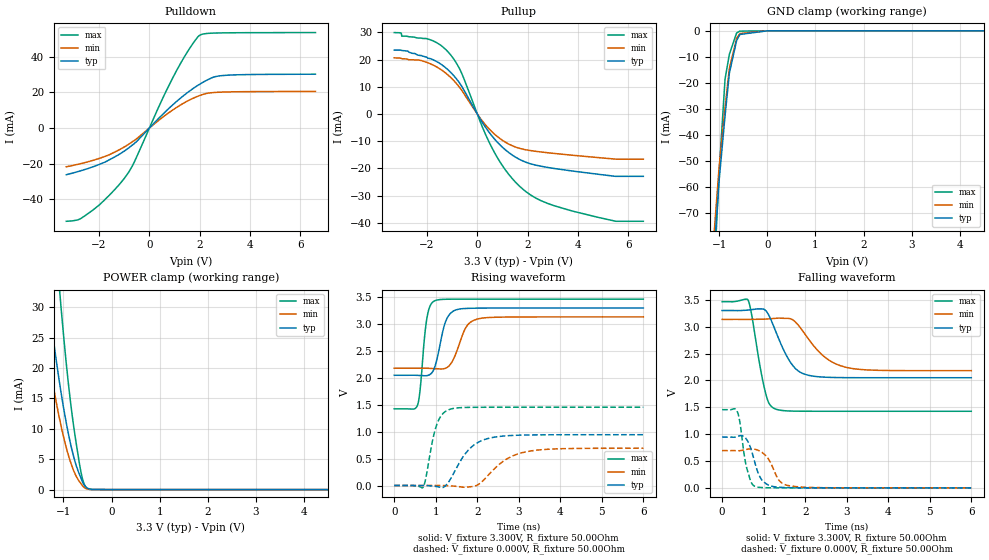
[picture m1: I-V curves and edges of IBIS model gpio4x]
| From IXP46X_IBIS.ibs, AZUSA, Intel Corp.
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[Model]   gpio4x
Model_type   I/O
Vinl = 800.000mV
Vinh = 2.000V
Vmeas = 1.500V
Cref = 0.000F
|   typ   min   max
C_comp   3.000pF   2.700pF   3.300pF
[Voltage Range]   3.300V   3.135V   3.465V
[Temperature Range]   25.0   110.0   -40.0
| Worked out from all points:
|   slope of the pulldown table from 0 to 0.495 V, typ, clamps not added: 68.7 ohm
|   slope of the pullup table from 0 to 0.495 V, typ, clamps not added: 70.3 ohm
|   POWER clamp passes 1 mA (typ) near -0.59 V on its own axis
|   falling waveform, V_fixture 3.300V, R_fixture 50.00Ohm: 20-80 % time 460ps typ, 667ps min, 278ps max; typ from 3.3 V to 2.05 V
|   rising waveform, V_fixture 3.300V, R_fixture 50.00Ohm: 20-80 % time 226ps typ, 291ps min, 146ps max; typ from 2.05 V to 3.3 V
|   rising waveform, V_fixture 0.000V, R_fixture 50.00Ohm: 20-80 % time 520ps typ, 669ps min, 242ps max; typ from 0 V to 0.944 V
|   falling waveform, V_fixture 0.000V, R_fixture 50.00Ohm: 20-80 % time 241ps typ, 274ps min, 183ps max; typ from 0.944 V to 0 V
[Pulldown]
|   Voltage   I(typ)   I(min)   I(max)
-3.3V     -26.23mA   -21.78mA   -52.39mA
-2.81V    -24.38mA   -20.3mA    -51.42mA
-2.245V   -21.81mA   -18.2mA    -46.09mA
-1.565V   -17.68mA   -14.82mA   -37.38mA
-910mV    -12.13mA   -9.924mA   -26.64mA
-605mV    -8.83mA    -7.087mA   -19.28mA
940mV     13.15mA    10.23mA    28.48mA
1.535V    20.1mA     15.3mA     43.29mA
1.99V     24.51mA    18.19mA    51.99mA
2.545V    28.53mA    19.9mA     53.28mA
2.875V    29.4mA     20.15mA    53.4mA
6.595V    30.22mA    20.54mA    53.58mA
[GND Clamp]
|   Voltage   I(typ)   I(min)   I(max)
-3.3V     -1.837A    -1.782A    -2.189A
-1.12V    -88.02mA   -80.79mA   -98.45mA
-1.005V   -57.96mA   -52.72mA   -55.07mA
-1V       -56.71mA   -51.74mA   -53.25mA
-880mV    -32.63mA   -29.48mA   -18.52mA
-790mV    -16.22mA   -14.39mA   -8.985mA
-640mV    -3.751mA   -2.926mA   -836.8uA
-575mV    -1.515mA   -1.11mA    -135.3uA
0V        -56.84nA   -17.58nA   -565.5pA
6.595V    0A         0A         0A
[Pullup]
|   Voltage   I(typ)   I(min)   I(max)
-3.3V     23.5mA     20.67mA    29.96mA
-1.775V   20.04mA    18.1mA     26.98mA
-1.055V   15.31mA    13.43mA    21.71mA
-630mV    10.36mA    8.892mA    15.17mA
215mV     -3.323mA   -2.738mA   -5.088mA
695mV     -9.323mA   -7.506mA   -14.38mA
1.25V     -14.19mA   -11.07mA   -22.21mA
1.945V    -17.79mA   -13.19mA   -28.66mA
2.78V     -19.63mA   -14.24mA   -32.84mA
3.825V    -21.04mA   -15.21mA   -35.82mA
5.505V    -22.94mA   -16.6mA    -39.47mA
6.595V    -22.94mA   -16.6mA    -39.47mA
[POWER Clamp]
|   Voltage   I(typ)   I(min)   I(max)
-3.3V     221.1mA    178.3mA    361mA
-1.495V   43.96mA    31.64mA    79.31mA
-1.32V    31.69mA    22.21mA    58.04mA
-1.2V     24.19mA    16.55mA    44.79mA
-1.08V    17.53mA    11.61mA    32.8mA
-1.045V   15.76mA    10.32mA    29.57mA
-910mV    9.707mA    6.02mA     18.41mA
-800mV    5.804mA    3.373mA    11.15mA
-640mV    2mA        1.037mA    3.043mA
-540mV    479.4uA    207uA      465.4uA
-395mV    31.37uA    12.42uA    6.173uA
6.595V    0A         0A         0A
[Ramp]
R_load = 50.00Ohm
|   typ   min   max
dV/dt_r   566.512mV/519.754ps 416.047mV/666.991ps 873.059mV/242.006ps
dV/dt_f   750.486mV/460.386ps 572.648mV/665.835ps   1.224V/277.588ps
[Falling Waveform]
V_fixture = 3.300V
V_fixture_min = 3.135V
V_fixture_max = 3.465V
R_fixture = 50.00Ohm
|   Time   V(typ)   V(min)   V(max)
0s        3.3V       3.135V     3.465V
630ps     3.309V     3.134V     3.485V
1.04ns    3.305V     3.14V      1.785V
1.13ns    3.203V     3.145V     1.572V
1.27ns    2.953V     3.154V     1.472V
1.66ns    2.32V      3.142V     1.429V
2.04ns    2.102V     2.812V     1.426V
2.51ns    2.058V     2.411V     1.425V
3.03ns    2.051V     2.235V     1.425V
6ns       2.049V     2.181V     1.425V
[Rising Waveform]
V_fixture = 3.300V
V_fixture_min = 3.135V
V_fixture_max = 3.465V
R_fixture = 50.00Ohm
|   Time   V(typ)   V(min)   V(max)
0s        2.049V     2.181V     1.425V
560ps     2.048V     2.181V     1.489V
620ps     2.045V     2.182V     1.755V
790ps     2.043V     2.18V      3.121V
980ps     2.211V     2.172V     3.436V
1.24ns    3.052V     2.181V     3.462V
1.51ns    3.27V      2.503V     3.465V
1.74ns    3.292V     2.955V     3.465V
2.06ns    3.298V     3.105V     3.465V
6ns       3.3V       3.135V     3.465V
[Rising Waveform]
V_fixture = 0.000V
V_fixture_min = 0.000V
V_fixture_max = 0.000V
R_fixture = 50.00Ohm
|   Time   V(typ)   V(min)   V(max)
0s        1.619uV    550.4nV    -9.718nV
690ps     406.1uV    94.12uV    -38.08mV
1.02ns    -18.89mV   352.9uV    1.121V
1.19ns    -31.72mV   -1.564mV   1.349V
1.35ns    112.8mV    -7.119mV   1.419V
1.8ns     670mV      -25.67mV   1.453V
2.34ns    888.7mV    254.3mV    1.455V
2.75ns    926.5mV    510.9mV    1.455V
3.31ns    940.3mV    645mV      1.455V
6ns       944.2mV    693.4mV    1.455V
[Falling Waveform]
V_fixture = 0.000V
V_fixture_min = 0.000V
V_fixture_max = 0.000V
R_fixture = 50.00Ohm
|   Time   V(typ)   V(min)   V(max)
0s        944.2mV    693.4mV    1.455V
370ps     956mV      691.5mV    1.411V
430ps     970.8mV    692mV      1.211V
590ps     901.1mV    715.4mV    378.4mV
700ps     710.9mV    726.4mV    105mV
820ps     383.6mV    712.8mV    19.15mV
1.07ns    71.73mV    583.6mV    2.709mV
1.36ns    12.48mV    151.9mV    457.5uV
1.58ns    4.985mV    44.71mV    122.8uV
6ns       1.619uV    550.4nV    -9.718nV
